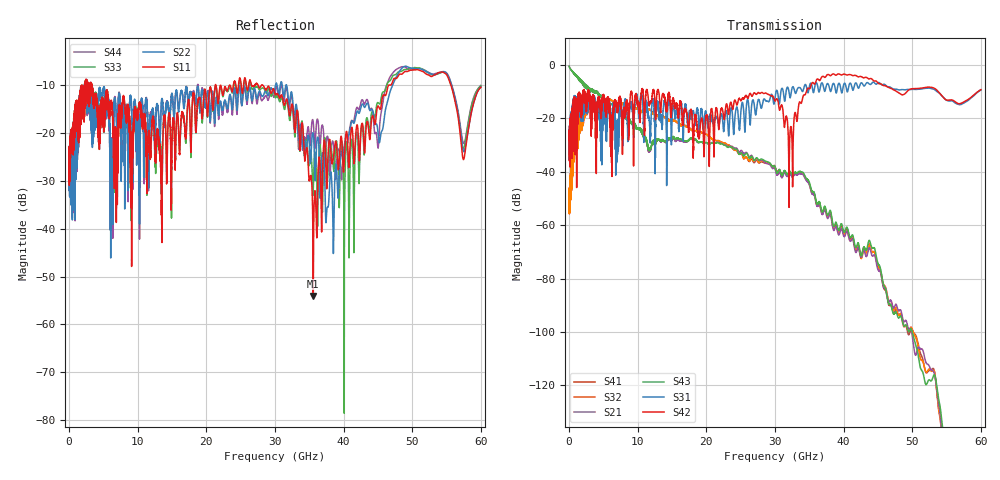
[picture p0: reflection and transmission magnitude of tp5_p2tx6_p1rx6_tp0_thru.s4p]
! 100G CR Analysis
! File: tp5_p2tx6_p1rx6_tp0_thru
! Description: 2m Cu Cable, OSFP, TP0-TP5
! Port Mapping
! Port1 -- P1RX6N
! Port2 -- P2TX6N
! Port3 -- P1RX6P
! Port4 -- P2TX6P
# GHz S MA R 50.00
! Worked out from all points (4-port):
!   6000 points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, 10 MHz to 60 GHz, reference 50 ohm
!   strongest paths, dB at 10 MHz, 15.01 GHz, 30.01 GHz, 45.01 GHz, 60 GHz:
!     S42: -28.2, -14.6, -13.5, -6.8, -9.3
!     S31: -27.9, -20.3, -12.3, -6.7, -9.4
!     S43: -0.5, -27.5, -38.2, -74.3, -173.5
!     S21: -0.5, -27.9, -39.0, -76.7, -166.7
!     S32: -46.8, -20.6, -38.3, -75.6, -172.4
!     S41: -46.6, -20.5, -38.1, -75.7, -169.2
!   lowest |S11| = -54.1 dB at 35.58 GHz (marker M1), VSWR 1.00, Z = 50.2 - j0.1 ohm
!   |S11| at or under -10 dB: 3.325 GHz to 21.29 GHz (17.97 GHz wide, 146 % of centre); 28.26 GHz to 46.54 GHz (18.27 GHz wide, 48.9 % of centre); 55.65 GHz to end of sweep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
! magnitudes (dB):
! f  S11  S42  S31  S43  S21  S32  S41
! 10 MHz  -24.0  -28.2  -27.9  -0.5  -0.5  -46.8  -46.6
! 6.03 GHz  -15.0  -30.7  -17.5  -14.9  -15.0  -12.9  -12.9
! 28.36 GHz  -10.2  -10.7  -12.9  -35.6  -36.1  -36.3  -36.6
! 32.31 GHz  -15.0  -23.2  -11.3  -40.3  -41.0  -40.6  -40.6
! 35.58 GHz  -54.1  -6.7  -10.3  -47.4  -48.3  -47.9  -47.8
! 45.88 GHz  -12.0  -7.7  -7.2  -82.8  -83.5  -82.6  -83.9
! 60 GHz  -10.4  -9.3  -9.4  -173.5  -166.7  -172.4  -169.2
